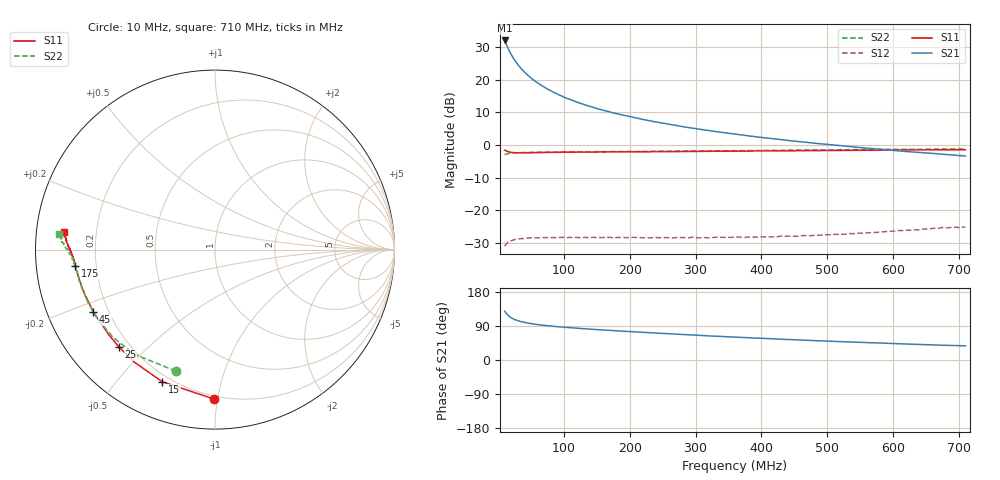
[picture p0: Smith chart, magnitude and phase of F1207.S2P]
!  POLYFET RF DEVICES
!  S PARAMETER FOR
!  F1207
!  VDS=12.5V IDS=400MA
!  APR 12TH  1996
# MHZ  S  MA  R  50.0000
!  FREQ  MAG[S11]  ANG  MAG[S21]  ANG  MAG[S12]  ANG	MAG[S22]  ANG
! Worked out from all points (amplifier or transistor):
!   141 points, 10 MHz to 710 MHz, reference 50 ohm
!   highest |S21| = 32.1 dB at 10 MHz (marker M1)
!   |S21| within 3 dB of that: start of sweep to 16.72 MHz
!   unconditionally stable (mu >= 1): 349.1 MHz to end of sweep
!   at 125 MHz: K = 0.42, MSG = 20.7 dB, |S12| = -28.5 dB
!   at 360 MHz: K = 1.01, MAG = 15.2 dB, |S12| = -28.3 dB
!   at 710 MHz: K = 1.12, MAG = 8.9 dB, |S12| = -25.2 dB
!   S11 on the Smith chart (normalised r, x): 10 MHz: 0.18, -0.98; 15 MHz: 0.17, -0.66; 25 MHz: 0.16, -0.41; 45 MHz: 0.14, -0.24; 175 MHz: 0.12, -0.06; 710 MHz: 0.08, +0.06
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10  0.8337 -90.2  40.38 128.6  0.02788 37.9  0.7113 -107.8
15  0.7926 -111.8  30.96 118.1  0.03225 29.7  0.7354 -127.4
20  0.7713 -125.5  24.56 111.3  0.03382 24.4  0.7491 -139.0
25  0.7622 -134.7  20.28 107.0  0.03518 20.9  0.7556 -146.7
30  0.7583 -141.2  17.26 103.9  0.03614 18.1  0.7623 -151.9
35  0.7561 -145.9  14.97 101.3  0.03639 16.0  0.7636 -155.8
40  0.7579 -149.7  13.23 99.3  0.03646 15.2  0.7676 -158.6
45  0.762 -152.8  11.84 97.5  0.03708 14.3  0.7684 -161.0
50  0.7611 -155.1  10.71 96.1  0.03749 13.8  0.7716 -162.7
60  0.7645 -159.1  9.01 93.6  0.03754 12.7  0.7734 -165.7
65  0.7669 -160.6  8.338 92.5  0.03744 12.4  0.7762 -166.7
75  0.7687 -163.0  7.25 90.5  0.03778 10.6  0.777 -168.4
85  0.7701 -165.1  6.41 88.8  0.0378 11.5  0.7775 -169.9
100  0.7746 -167.3  5.458 86.6  0.03816 10.6  0.7809 -171.7
130  0.7768 -170.6  4.2 82.6  0.03799 12.1  0.7858 -173.5
150  0.7819 -172.0  3.637 80.2  0.03766 12.7  0.7917 -174.6
175  0.7843 -173.4  3.111 77.5  0.03735 13.7  0.7921 -175.3
245  0.7899 -176.2  2.211 70.6  0.03754 17.6  0.8003 -177.5
360  0.8036 -179.0  1.468 60.4  0.03845 25.9  0.8172 -179.5
480  0.8202 178.0  1.066 51.2  0.04091 38.3  0.8359 178.8
595  0.8343 175.7  0.8366 43.6  0.04702 49.0  0.8569 176.6
710  0.8459 173.5  0.6767 37.3  0.05465 53.9  0.8712 174.4
